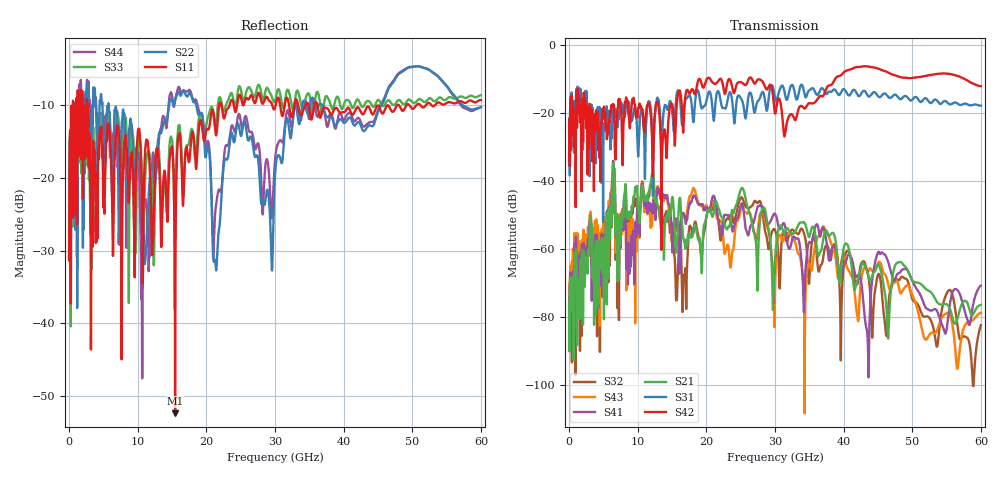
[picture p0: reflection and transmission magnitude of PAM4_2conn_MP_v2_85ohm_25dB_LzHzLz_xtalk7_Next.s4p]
! Info: Touchstone file created by Circ.  Input file=FAB50GbE_2conn_Midplane_Examax_Topo2_v2_85ohm_25dB_LzHzLz.circ
# Hz S RI R 50
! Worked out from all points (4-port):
!   6000 points, 10 MHz to 60 GHz, reference 50 ohm
!   strongest paths, dB at 10 MHz, 15.01 GHz, 30.01 GHz, 45.01 GHz, 60 GHz:
!     S42: -34.0, -17.4, -20.2, -7.0, -12.1
!     S31: -33.7, -19.3, -15.7, -15.1, -17.9
!     S21: -75.8, -44.9, -63.0, -64.5, -76.5
!     S41: -88.8, -59.0, -49.8, -61.1, -70.9
!     S43: -77.5, -56.1, -72.0, -64.3, -78.9
!     S32: -81.1, -54.0, -54.6, -67.6, -82.5
!   lowest |S11| = -52.4 dB at 15.45 GHz (marker M1), VSWR 1.00, Z = 49.8 + j0.104 ohm
!   |S11| at or under -10 dB: 2.8 GHz to 21.89 GHz (19.09 GHz wide, 155 % of centre); 22.21 GHz to 23.39 GHz (1.178 GHz wide, 5.17 % of centre); 36.17 GHz to 47.81 GHz (11.64 GHz wide, 27.7 % of centre)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
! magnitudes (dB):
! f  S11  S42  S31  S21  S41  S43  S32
! 10 MHz  -31.3  -34.0  -33.7  -75.8  -88.8  -77.5  -81.1
! 6.4 GHz  -30.7  -17.8  -20.8  -37.6  -34.4  -34.4  -37.7
! 15.45 GHz  -52.4  -28.3  -20.0  -57.1  -53.0  -52.7  -65.0
! 25.13 GHz  -9.3  -11.0  -16.0  -42.2  -46.7  -47.5  -44.8
! 29.75 GHz  -10.5  -15.6  -12.8  -75.6  -50.0  -68.2  -54.3
! 43.35 GHz  -10.3  -6.3  -14.4  -66.1  -83.6  -66.0  -66.0
! 60 GHz  -9.3  -12.1  -17.9  -76.5  -70.9  -78.9  -82.5
